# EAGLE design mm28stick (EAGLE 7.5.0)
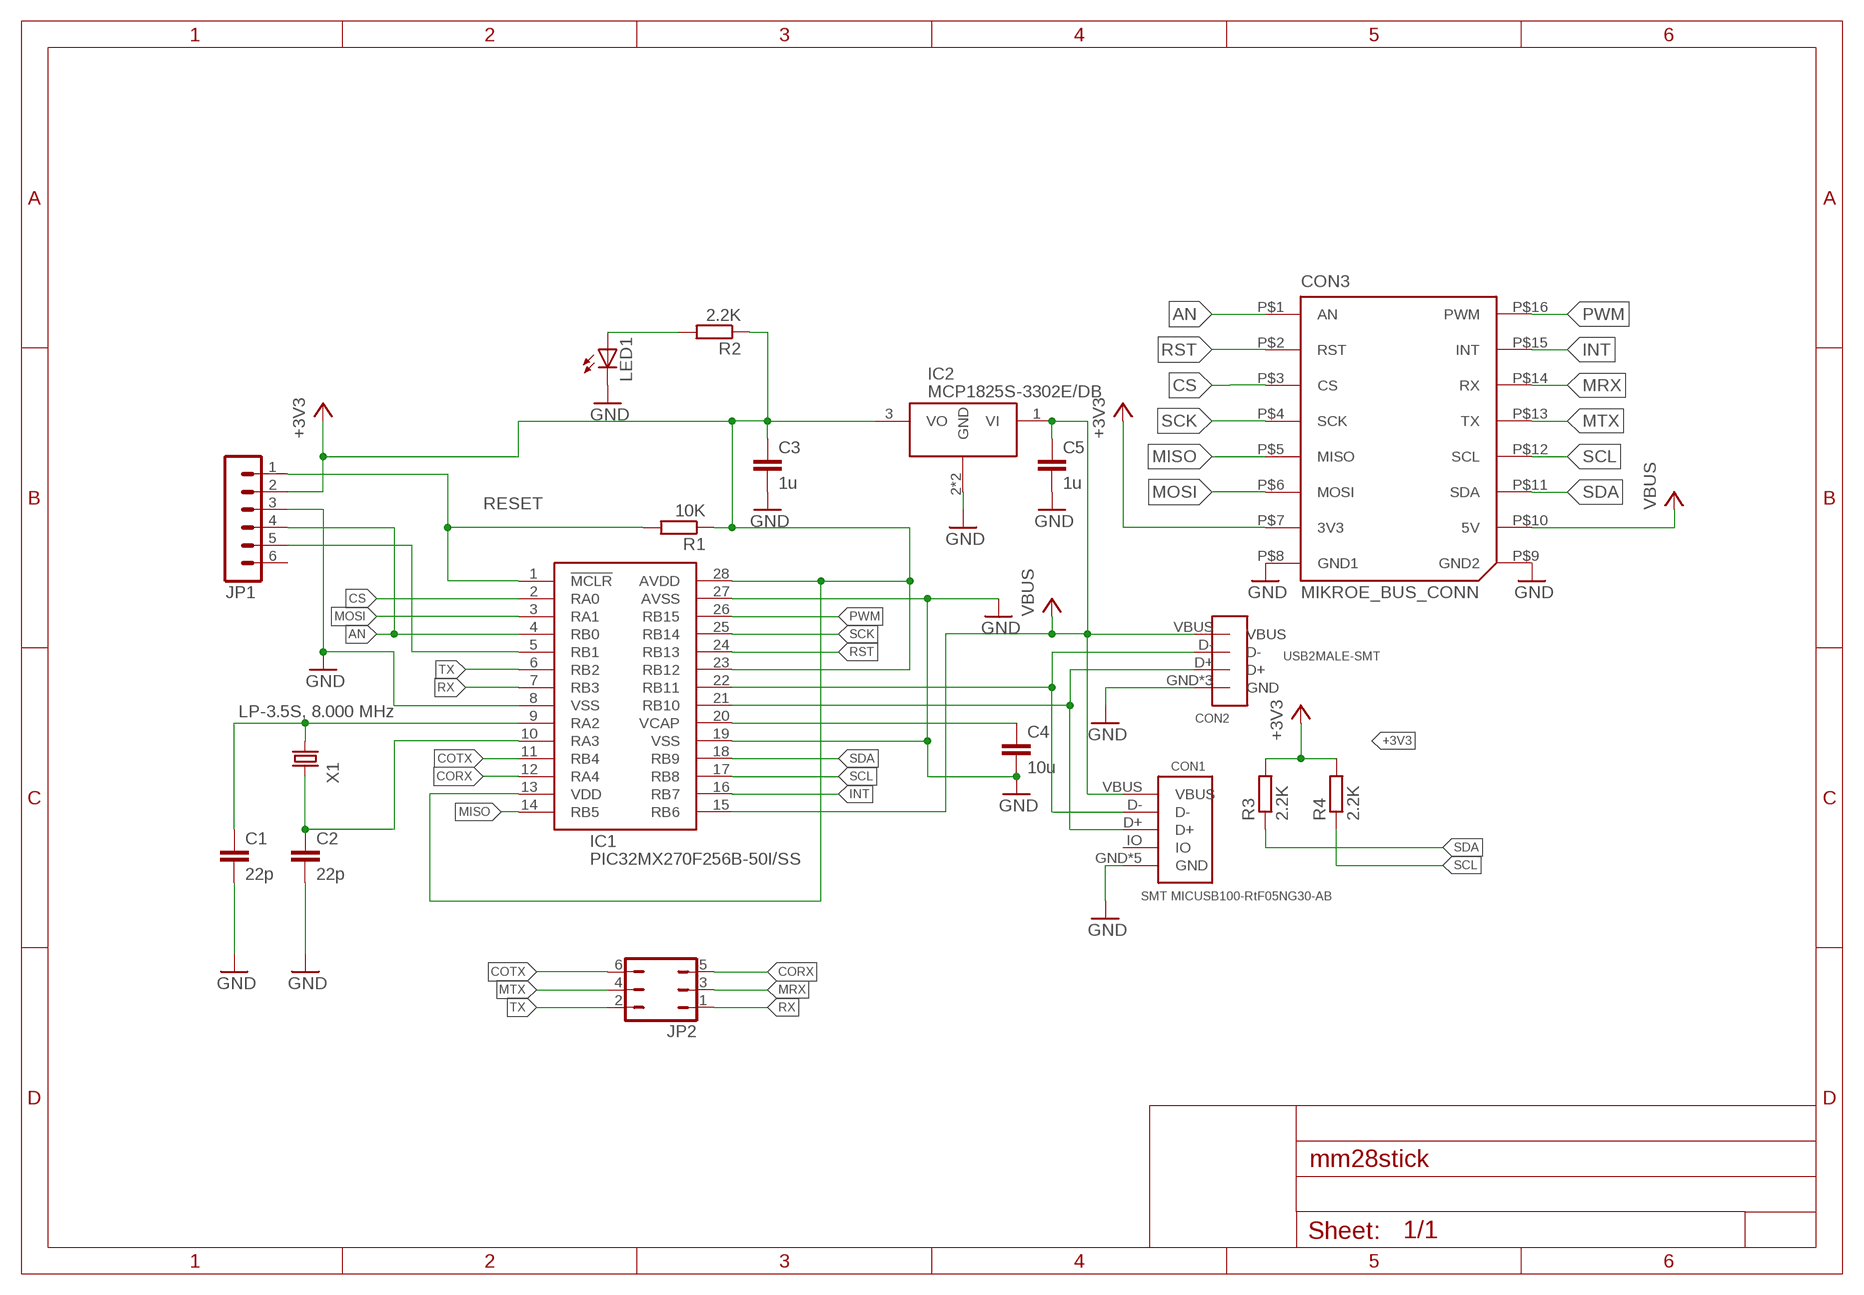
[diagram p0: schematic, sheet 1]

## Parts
C1  22p  C-EUC0805  [C0805]
C2  22p  C-EUC0805  [C0805]
C3  1u  C-EUC0805  [C0805]
C4  10u  C-EUC1210  [C1210]
C5  1u  C-EUC0805  [C0805]
CON1  SMT MICUSB100-RtF05NG30-AB  USB-MIC-SMT  [USB-MIC-SMT]
CON2  USB2MALE-SMT  [USB2MALE-SMT]
CON3  MIKROE_BUS_CONN  [MIKROBUS_HOST_CONN]
IC1  PIC32MX270F256B-50I/SS  MICROMITE28SS  [SSOP28]
IC2  MCP1825S-3302E/DB  MCP1825S-XX02E/DB  [SOT223]
JP1  MA06-1MA06-1B  [MA06-1B]
JP2  JP3Q  [JP3Q]
LED1  LEDSML1206  [SML1206]
R1  10K  R-EU_R0805  [R0805]
R2  2.2K  R-EU_R0805  [R0805]
R3  2.2K  R-EU_R0805  [R0805]
R4  2.2K  R-EU_R0805  [R0805]
X1  LP-3.5S, 8.000 MHz  CRYSTALS-NOGND-4-HSMX  [HC49-4-HSMX]

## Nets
+3V3: C3.1 CON3.P$7(3V3) IC1.13(VDD) IC1.23(RB12) IC1.28(AVDD) IC2.3(VO) JP1.2 R1.1 R2.1 R3.2 R4.2
AN: CON3.P$1(AN) IC1.4(RB0) JP1.4
CORX: IC1.12(RA4) JP2.5
COTX: IC1.11(RB4) JP2.6
CS: CON3.P$3(CS) IC1.2(RA0)
GND: C1.2 C2.2 C3.2 C4.2 C5.2 CON1.GND CON1.P$1(GND) CON1.P$2(GND) CON1.P$3(GND) CON1.P$4(GND) CON2.GND CON2.P$1(GND) CON2.P$2(GND) CON3.P$8(GND1) CON3.P$9(GND2) IC1.8(VSS) IC1.19(VSS) IC1.27(AVSS) IC2.2(GND) IC2.4(GND) JP1.3 LED1.C
INT: CON3.P$15(INT) IC1.16(RB7)
MISO: CON3.P$5(MISO) IC1.14(RB5)
MOSI: CON3.P$6(MOSI) IC1.3(RA1)
MRX: CON3.P$14(RX) JP2.3
MTX: CON3.P$13(TX) JP2.4
N$1: CON1.D- CON2.D- IC1.22(RB11)
N$2: CON1.D+ CON2.D+ IC1.21(RB10)
N$3: IC1.5(RB1) JP1.5
N$4: C4.1 IC1.20(VCAP)
N$5: C1.1 IC1.9(RA2) X1.2
N$7: C2.1 IC1.10(RA3) X1.1
N$9: LED1.A R2.2
PWM: CON3.P$16(PWM) IC1.26(RB15)
RESET: IC1.1(!MCLR!) JP1.1 R1.2
RST: CON3.P$2(RST) IC1.24(RB13)
RX: IC1.7(RB3) JP2.1
SCK: CON3.P$4(SCK) IC1.25(RB14)
SCL: CON3.P$12(SCL) IC1.17(RB8) R4.1
SDA: CON3.P$11(SDA) IC1.18(RB9) R3.1
TX: IC1.6(RB2) JP2.2
VCC: C5.1 CON1.VBUS CON2.VBUS CON3.P$10(5V) IC1.15(RB6) IC2.1(VI) ; supply symbol labelled VBUS
Unconnected: CON1.IO JP1.6

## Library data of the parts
C1-C5 = kando2:C-EU: CAPACITOR, European symbol
CON1 = drk:USB-MIC-SMT
CON2 = drk:USB2MALE-SMT
CON3 = mikrobus_lib:MIKROE_BUS_CONN
IC1 = z01:MICROMITE28: 28 pin MicroMite
IC2 = z01:MCP1825S-XX02E/: MCP1825S 500 mA, Low Voltage, Low Quiescent Current LDO Regulator
JP1 = kando2:MA06-1: PIN HEADER
JP2 = mm28stick:JP3Q: JUMPER
LED1 = led:LED: LED
R1-R4 = kando2:R-EU_: RESISTOR, European symbol
X1 = IQD-Frequency-Products:CRYSTALS-NOGND: CRYSTALS CAN NOT GROUNDED

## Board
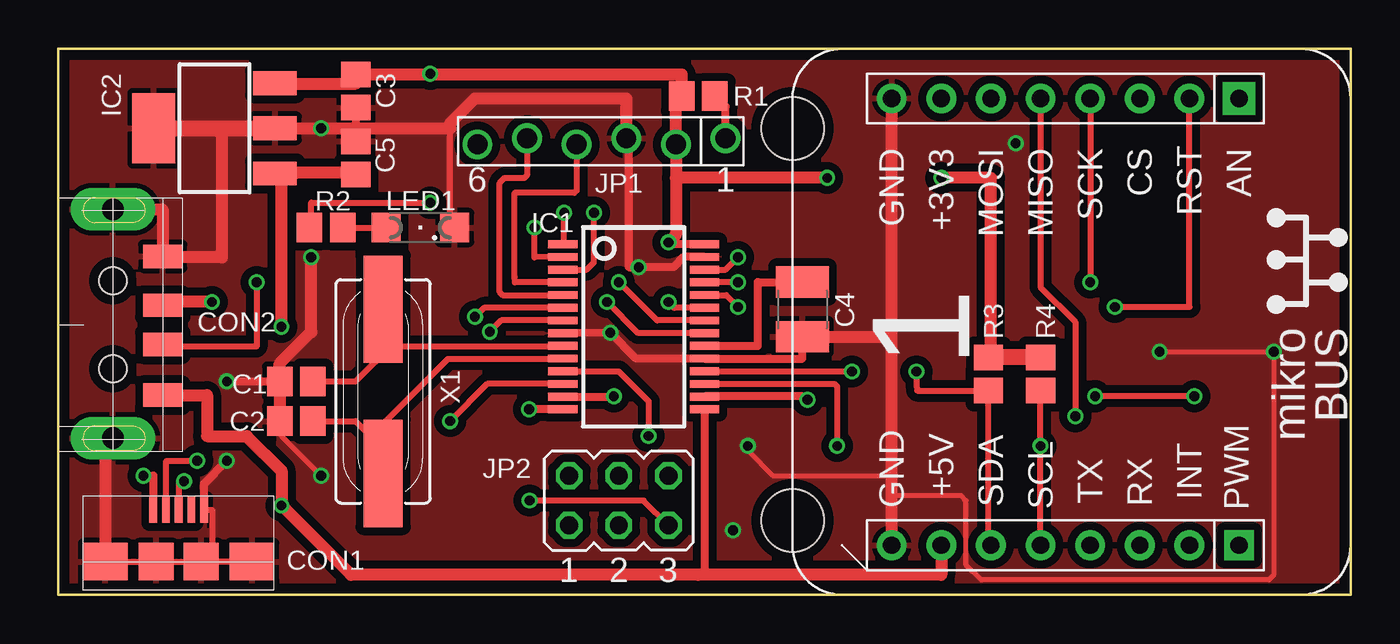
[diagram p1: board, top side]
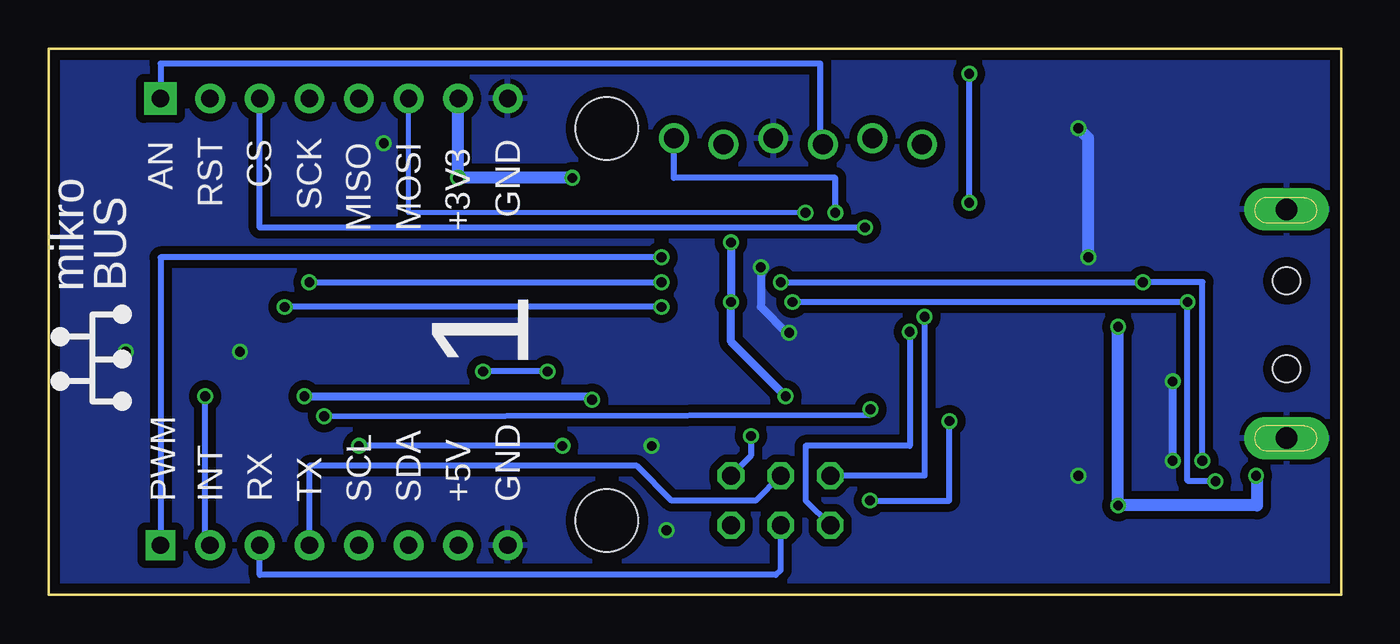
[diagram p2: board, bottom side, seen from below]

Size 66.17 x 27.94 mm. Coordinates in mm from the lower left corner, seen from the top.
Outline: 66.17,27.94 0,27.94 0,0 66.17,0 66.17,27.94
Copper layers (1*16): Top 0.035mm / dielectric 1.6mm / Bottom 0.035mm
Design rules "Elecrow_2-layer_PCB_eagle_rule *": minimum track width 8mil, minimum drill 0.5mm, track to track 8mil, track to pad 8mil, pad to pad 8mil, via to via 8mil, smd to smd 0mil, copper to edge 20mil, drill to drill 10mil, minimum pad ring 6mil, minimum via ring 6mil, stop-mask expansion 0mil, vias tented up to drill 100mil, thermal gap 10mil
Holes 3.2 mm at 37.59,23.88 37.59,3.81

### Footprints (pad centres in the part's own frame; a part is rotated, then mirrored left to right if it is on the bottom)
C0805 = smd 1.3 x 1.5: 1 -0.85,0; 2 0.85,0
C1210 = smd 1.6 x 2.7: 1 -1.4,0; 2 1.4,0
USB-MIC-SMT = smd 0.4 x 1.35: D+ 4.9,4.1; D- 4.25,4.1; GND 6.2,4.1; IO 5.55,4.1; VBUS 3.6,4.1 | smd 1.8 x 1.9: P$1 3.75,1.45; P$2 6.05,1.45 | smd 2.3 x 1.9: P$3 1.15,1.45; P$4 8.65,1.45
USB2MALE-SMT = smd 1.2 x 2: D+ 5.5,5.35; D- 7.5,5.35; GND 3,5.35; VBUS 10.1,5.35 | drill 1.1 pad 2.184 long: P$1 0.6,2.8; P$2 12.3,2.8 | hole 1.4: 4.25,2.8; 8.75,2.8
MIKROBUS_HOST_CONN = drill 0.889 pad 1.676 square: P$1 0,0 | drill 0.889 pad 1.524: P$2 0,-2.54; P$3 0,-5.08; P$4 0,-7.62; P$5 0,-10.16; P$6 0,-12.7; P$7 0,-15.24; P$8 0,-17.78; P$9 22.86,-17.78; P$10 22.86,-15.24; P$11 22.86,-12.7; P$12 22.86,-10.16; P$13 22.86,-7.62; P$14 22.86,-5.08; P$15 22.86,-2.54 | drill 0.889 pad 1.524 square: P$16 22.86,0
SSOP28 = smd 0.4 x 1.5: 1 -4.225,-3.625; 2 -3.575,-3.625; 3 -2.925,-3.625; 4 -2.275,-3.625; 5 -1.625,-3.625; 6 -0.975,-3.625; 7 -0.325,-3.625; 8 0.325,-3.625; 9 0.975,-3.625; 10 1.625,-3.625; 11 2.275,-3.625; 12 2.925,-3.625; 13 3.575,-3.625; 14 4.225,-3.625; 15 4.225,3.625; 16 3.575,3.625; 17 2.925,3.625; 18 2.275,3.625; 19 1.625,3.625; 20 0.975,3.625; 21 0.325,3.625; 22 -0.325,3.625; 23 -0.975,3.625; 24 -1.625,3.625; 25 -2.275,3.625; 26 -2.925,3.625; 27 -3.575,3.625; 28 -4.225,3.625
SOT223 = smd 1.219 x 2.235: 1 -2.311,-3.099; 2 0,-3.099; 3 2.311,-3.099 | smd 3.6 x 2.2: 4 0,3.099
MA06-1B = drill 1.016: 1 -6.35,0; 2 -3.81,0.318; 3 -1.27,0; 4 1.27,0.318; 5 3.81,0; 6 6.35,0.318
JP3Q = drill 0.914 octagon: 1 -2.54,-1.27; 2 -2.54,1.27; 3 0,-1.27; 4 0,1.27; 5 2.54,-1.27; 6 2.54,1.27
SML1206 = smd 1.5 x 1.5: A 1.75,0; C -1.75,0
R0805 = smd 1.3 x 1.5: 1 -0.85,0; 2 0.85,0
HC49-4-HSMX = smd 5.5 x 2: 1 -4.2,0; 2 4.2,0

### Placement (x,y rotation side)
C1  12.19,10.92 180 top
C2  12.19,8.89 180 top
C3  15.24,25.78 270 top
C4  38.1,14.61 270 top
C5  15.24,22.35 90 top
CON1  1.27,0.25 0 top
CON2  0,20.32 270 top
CON3  60.45,25.4 270 top
IC1  29.46,13.72 270 top
IC2  8,23.88 90 top
JP1  27.81,23.37 180 top
JP2  28.7,4.83 0 top
LED1  18.54,18.8 180 top
R1  32.77,25.53 0 top
R2  13.72,18.8 0 top
R3  47.62,11.3 90 top
R4  50.29,11.3 90 top
X1  16.64,10.41 90 top

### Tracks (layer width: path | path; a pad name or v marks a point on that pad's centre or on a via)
+3V3  (via drill 0.5 pad 0.81)
  Top 0.305: 50.33,12.19 R4.2 | IC1.23 31.54,14.69 v31.24,14.99 | 28.43,10.14 v28.45,10.16 | 15.24,26.16 C3.1 | 19.05,26.63 v19.05,26.67 | R2.1 12.95,18.8 12.95,20.07 v19.05,20.07
  Top 0.406: IC2.3 11.86,26.16 | 31.62,25.23 R1.1 | IC1.28 31.34,17.94 v31.24,18.03 | IC1.13 28.43,10.14
  Top 0.61: 31.62,25.23 JP1.2 31.62,21.34 | 31.62,21.34 31.62,18.41 v31.24,18.03 | v39.37,21.34 31.62,21.34 | 11.86,26.16 15.24,26.16 | C3.1 19.05,26.63 31.92,26.63 R1.1 | R3.2 47.75,12.15 47.75,21.34 v45.21,21.34
  Top 0.813: R4.2 R3.2
  Bottom 0.305: v19.05,20.07 v19.05,26.67
  Bottom 0.406: v31.24,18.03 v31.24,14.99 31.24,12.95 v28.45,10.16
  Bottom 0.61: v39.37,21.34 v45.21,21.34 CON3.P$7
AN
  Top 0.305: IC1.4 23.38,15.99 23.37,16.26 23.37,20.57 26.42,20.57 26.54,20.7 JP1.4
  Bottom 0.305: 26.67,23.18 26.67,27.18 60.45,27.18 CON3.P$1
  Bottom 0.406: JP1.4 26.67,23.18
CORX  (via drill 0.5 pad 0.81)
  Top 0.305: JP2.5 29.97,4.83 v24.13,4.83 | IC1.12 21.97,10.79 v20.07,8.89
  Bottom 0.305: v24.13,4.83 20.07,4.83 v20.07,8.89
COTX  (via drill 0.5 pad 0.81)
  Top 0.305: IC1.11 28.69,11.44 30.23,9.91 v30.23,8.13
  Bottom 0.305: v30.23,8.13 30.23,7.11 JP2.6
CS  (via drill 0.5 pad 0.81)
  Top 0.305: IC1.2 24.38,17.27 v24.38,18.8
  Bottom 0.305: v24.38,18.8 55.37,18.8 CON3.P$3
GND  (via drill 0.5 pad 0.81)
  Top 0.254: 42.67,13.21 42.67,14.48 | v13.46,6.1 11.43,8.13 11.43,8.8 C2.2 | v56.39,12.45 v62.23,12.45 62.23,1.02 61.98,0.76 47.24,0.76 46.48,1.52 46.48,4.83 46.23,5.08 42.67,5.08 | v35.31,7.62 35.31,7.37 36.58,6.1 42.67,6.1
  Top 0.305: LED1.C 20.07,18.8 20.07,23.88 | CON1.P$4 7.87,1.7 | 7.87,1.7 CON1.P$2 CON1.P$1 CON1.P$3 | CON1.GND 7.87,4.35 7.87,1.7
  Top 0.406: C4.2 38.1,12.09 IC1.19 29.59,12.09 v28.27,13.41 IC1.8 | 14.9,23.2 C5.2 15.24,23.62 15.49,23.88 15.24,23.88 C3.2 | 6.1,23.88 IC2.4 | JP1.3 29.21,23.24 29.21,16.76 v29.72,16.76 31.5,16.76 32.02,17.29 IC1.27 | 4.83,22.61 4.83,23.88 8.13,23.88 8.13,23.62 8.38,23.62 | v8.64,6.86 7.47,5.69 CON1.GND | v8.64,10.92 C1.2
  Top 0.61: CON3.P$9 42.67,5.08 42.67,6.1 42.67,14.48 CON3.P$8 | C4.2 42.67,13.21 | C2.2 C1.2 11.34,11.85 12.95,13.46 v12.95,17.27 | IC2.2 v13.46,23.88 15.24,23.88 | 15.49,23.88 20.07,23.88 20.07,24.13 21.34,25.4 29.08,25.4 JP1.3 | 8.38,23.62 8.38,17.27 5.35,17.27 CON2.GND 5.35,19.72 CON2.P$1 | CON2.P$2 2.42,8.02 CON1.P$3
  Top 0.813: 4.83,23.88 6.1,23.88 IC2.2
  Bottom 0.406: v29.72,16.76 29.72,14.73 28.4,13.41 v28.27,13.41 | v8.64,6.86 v8.64,10.92
  Bottom 0.61: v12.95,17.27 12.95,23.37 v13.46,23.88
  other vias: 49.02,23.11 34.54,3.3
  pour Bottom (isolate 0.406): 0,27.94 66.04,27.94 66.04,0 0,0
  pour Top (isolate 0.406): 0,27.94 66.04,27.94 66.04,0 0,0
INT  (via drill 0.5 pad 0.81)
  Top 0.305: v58.17,10.16 v53.09,10.16
  Top 0.406: v38.35,9.98 38.35,9.91 38.1,10.16 33.11,10.16 IC1.16
  Bottom 0.305: CON3.P$15 58.17,2.79 v58.17,10.16
  Bottom 0.406: v53.09,10.16 38.61,10.16 38.35,9.91 v38.35,9.98
MISO  (via drill 0.5 pad 0.81)
  Top 0.305: CON3.P$5 50.29,15.75 52.07,13.97 v52.07,9.14
  Top 0.406: IC1.14 v24.1,9.49
  Bottom 0.305: v52.07,9.14 24.1,9.22 v24.1,9.49
MOSI  (via drill 0.5 pad 0.81)
  Top 0.305: IC1.3 27.05,16.64 27.43,17.02 v27.43,19.56
  Bottom 0.254: v27.43,19.56 47.75,19.56 CON3.P$6
MRX
  Bottom 0.305: JP2.3 28.7,1.27 28.96,1.02 55.37,1.02 CON3.P$14
MTX
  Bottom 0.305: JP2.4 29.97,4.83 34.29,4.83 36.07,6.6 52.83,6.6 CON3.P$13
N$1  (via drill 0.5 pad 0.81)
  Top 0.305: IC1.22 30.66,14.05 v28.7,16 | v10.16,16 10.16,12.7 5.35,12.7 | v7.11,6.86 5.54,6.86 5.54,4.35 CON1.D-
  Top 0.61: 5.35,12.7 CON2.D-
  Bottom 0.305: v28.7,16 v10.16,16 7.11,16 v7.11,6.86
N$2  (via drill 0.5 pad 0.81)
  Top 0.305: IC1.21 29.69,13.39 v28.1,14.99 | CON1.D+ 6.19,4.35 6.19,5.68 6.35,5.84 v6.44,5.81
  Top 0.61: v7.87,14.99 5.35,14.99 CON2.D+
  Bottom 0.305: v28.1,14.99 v7.87,14.99 7.87,5.84 6.48,5.84
  Bottom 0.406: 6.48,5.84 v6.44,5.81
N$3
  Top 0.305: JP1.5 24,21.46 23.88,21.34 22.86,21.34 22.61,21.08 22.61,15.49 22.76,15.34 IC1.5
N$4
  Top 0.406: IC1.20 35.81,12.74 35.81,16 C4.1
N$5
  Top 0.305: IC1.9 25.8,12.7 17.27,12.7 17.14,12.84 | 17.14,12.84 X1.2 | C1.1 15.22,10.92 17.14,12.84
N$7
  Top 0.305: IC1.10 25.81,12.07 19.94,12.07 16.76,8.89 16.76,7.37 | 16.64,5.71 16.51,5.84 16.51,6.09 X1.1 16.76,6.34 16.76,7.37 | C2.1 15.24,8.89 16.76,7.37
N$9
  Top 0.305: R2.2 LED1.A
PWM  (via drill 0.5 pad 0.81)
  Top 0.305: IC1.26 34.17,16.64 v34.8,17.27
  Bottom 0.305: CON3.P$16 60.45,17.27 v34.8,17.27
RESET  (via drill 0.5 pad 0.81)
  Top 0.305: IC1.1 25.91,17.94 v25.91,19.56
  Top 0.406: JP1.1 34.16,24.98 R1.2
  Bottom 0.305: v25.91,19.56 25.91,21.34 34.16,21.34 JP1.1
RST  (via drill 0.5 pad 0.81)
  Top 0.305: v54.1,14.73 57.91,14.73 CON3.P$2 | IC1.24 34.19,15.34 v34.8,14.73
  Bottom 0.305: v34.8,14.73 v54.1,14.73
RX  (via drill 0.5 pad 0.81)
  Top 0.305: IC1.7 22.68,14.04 v22.1,13.46
  Bottom 0.305: v22.1,13.46 22.1,7.62 27.43,7.62 27.43,4.83 JP2.1
SCK  (via drill 0.5 pad 0.81)
  Top 0.305: CON3.P$4 v52.83,16 | v34.8,16 IC1.25
  Bottom 0.305: v52.83,16 v34.8,16
SCL  (via drill 0.5 pad 0.81)
  Top 0.305: CON3.P$12 v50.29,7.62 R4.1 | IC1.17 39.75,10.79 39.88,10.67 v39.88,7.62
  Bottom 0.305: v39.88,7.62 v50.29,7.62
SDA  (via drill 0.5 pad 0.81)
  Top 0.254: CON3.P$11 47.62,2.67
  Top 0.305: 47.62,2.67 R3.1 43.98,10.45 43.94,10.67 v43.94,11.43 | IC1.18 33.1,11.43 v40.64,11.43
  Bottom 0.305: v40.64,11.43 v43.94,11.43
TX  (via drill 0.5 pad 0.81)
  Top 0.305: IC1.6 21.8,14.69 v21.34,14.22
  Bottom 0.305: v21.34,14.22 21.34,6.1 JP2.2
VCC  (via drill 0.5 pad 0.81)
  Top 0.406: C5.1 15.05,21.59 | IC2.1 11.63,21.59 12.19,21.59 11.61,21.51 | IC1.15 33.09,1.08 32.77,1.02 | v4.37,6.1 4.87,6.1 CON1.VBUS
  Top 0.61: 15.05,21.59 12.19,21.59 | CON3.P$10 45.21,1.02 32.77,1.02 14.99,1.02 v11.43,4.57 11.43,6.35 9.65,8.13 7.62,8.13 7.62,10.22 CON2.VBUS | v11.43,13.72 11.43,21.59 11.61,21.51
  Bottom 0.61: v4.37,6.1 4.32,6.1 4.32,4.57 v11.43,4.57 v11.43,13.72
